(* Logix 5000 AddOnInstructionDefinition export Banner_QS18E_Param_v3; software revision 30.00; part 3 of 3 *)
(* tags used below, declared in another part *)
   QS18E : Banner_QS18E_v3;
   Port_Data : Banner_IOL_Port_v2;
   Port : DINT;
   Local_Control : DINT;
   Command_Being_Processed : BOOL;
   Update_Archive : BOOL;
   Index_Write_Inprocess : INT;
   Inprocess_Index : DINT;
(* Banner_QS18E_Param_v3, continued *)

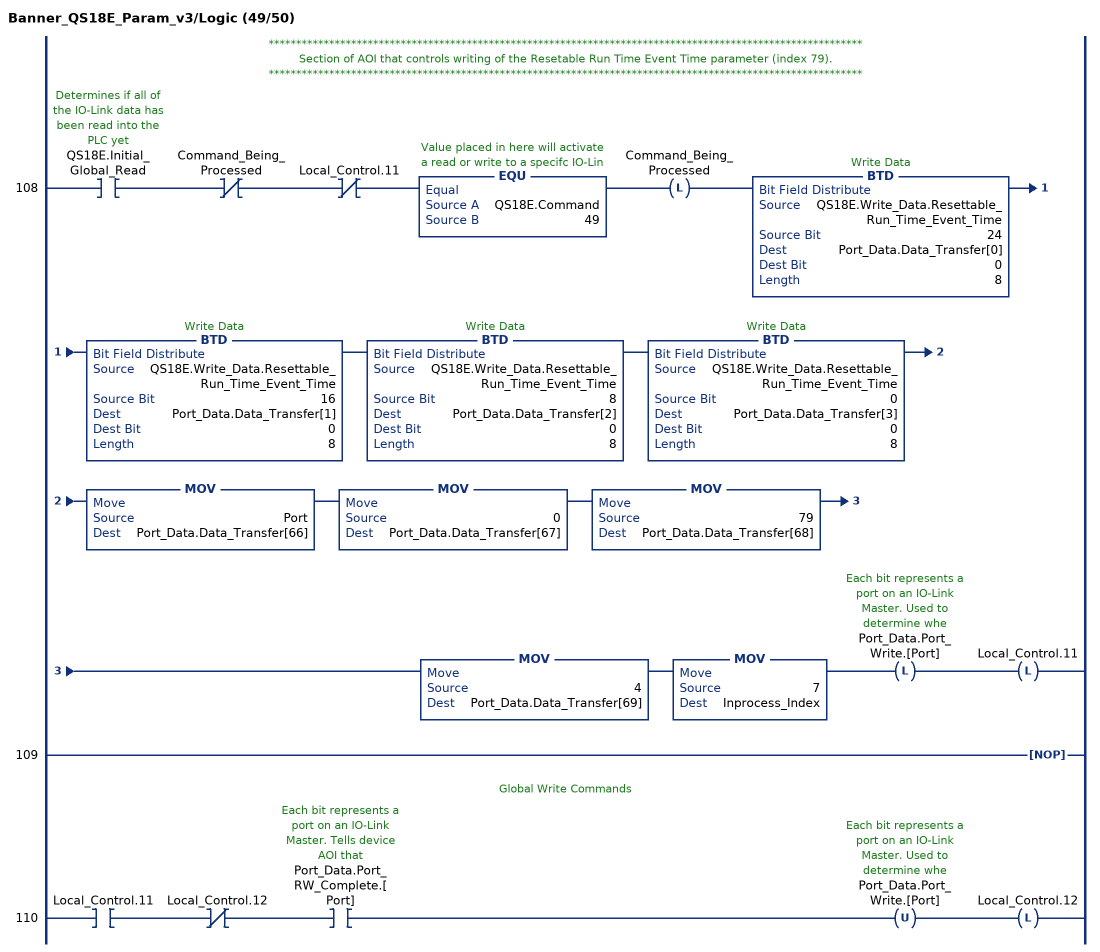
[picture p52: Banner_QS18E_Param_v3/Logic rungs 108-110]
   // ************************************************************************************************************
   // Section of AOI that controls writing of the Resetable Run Time Event Time parameter (index 79).
   // ************************************************************************************************************
   108: XIC(QS18E.Initial_Global_Read)XIO(Command_Being_Processed)XIO(Local_Control.11)EQU(QS18E.Command,49)OTL(Command_Being_Processed)BTD(QS18E.Write_Data.Resettable_Run_Time_Event_Time,24,Port_Data.Data_Transfer[0],0,8)BTD(QS18E.Write_Data.Resettable_Run_Time_Event_Time,16,Port_Data.Data_Transfer[1],0,8)BTD(QS18E.Write_Data.Resettable_Run_Time_Event_Time,8,Port_Data.Data_Transfer[2],0,8)BTD(QS18E.Write_Data.Resettable_Run_Time_Event_Time,0,Port_Data.Data_Transfer[3],0,8)MOV(Port,Port_Data.Data_Transfer[66])MOV(0,Port_Data.Data_Transfer[67])MOV(79,Port_Data.Data_Transfer[68])MOV(4,Port_Data.Data_Transfer[69])MOV(7,Inprocess_Index)OTL(Port_Data.Port_Write.[Port])OTL(Local_Control.11);
   109: NOP();
   // Global Write Commands
   110: XIC(Local_Control.11)XIO(Local_Control.12)XIC(Port_Data.Port_RW_Complete.[Port])OTU(Port_Data.Port_Write.[Port])OTL(Local_Control.12);
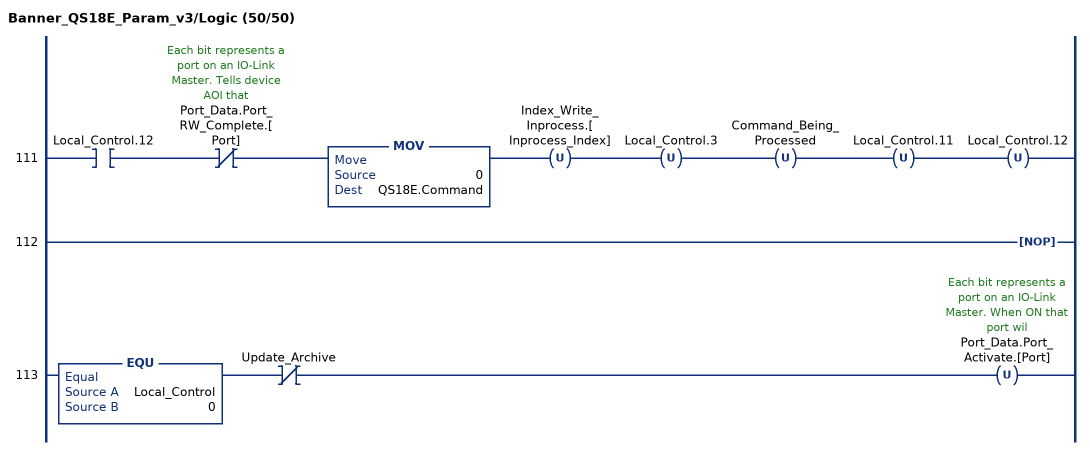
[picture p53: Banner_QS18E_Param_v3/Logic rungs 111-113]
   111: XIC(Local_Control.12)XIO(Port_Data.Port_RW_Complete.[Port])MOV(0,QS18E.Command)OTU(Index_Write_Inprocess.[Inprocess_Index])OTU(Local_Control.3)OTU(Command_Being_Processed)OTU(Local_Control.11)OTU(Local_Control.12);
   112: NOP();
   113: EQU(Local_Control,0)XIO(Update_Archive)OTU(Port_Data.Port_Activate.[Port]);
END_ROUTINE
END_ADD_ON_INSTRUCTION
